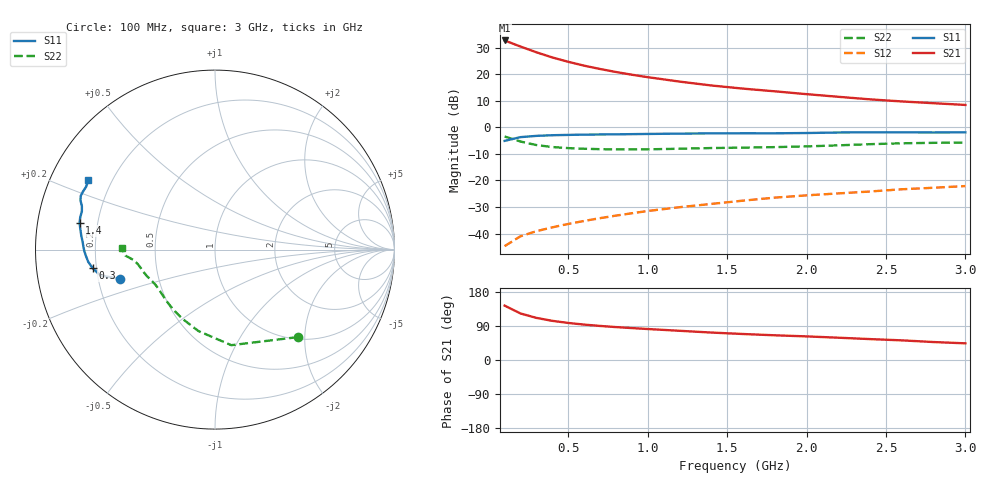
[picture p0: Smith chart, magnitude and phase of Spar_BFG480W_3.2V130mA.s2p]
! Filename: 3_2130BFG480.001
! Title: BFG480W
! Bias: Vce=3.2V; Ic=130mA
! Company: NXP Semiconductors NL
! User: Quality&Reliability T&D
! Measure time: 10 Nov 1999 / 11:58:35
#  MHz  S  MA  R 50
! Freq  S11  S21  S12  S22  :
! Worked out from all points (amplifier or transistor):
!   20 points, 100 MHz to 3 GHz, reference 50 ohm
!   highest |S21| = 32.7 dB at 100 MHz (marker M1)
!   |S21| within 3 dB of that: start of sweep to 232.7 MHz
!   unconditionally stable (mu >= 1): 528.6 MHz to end of sweep
!   at 400 MHz: K = 0.92, MSG = 31.9 dB, |S12| = -37.6 dB
!   at 1.2 GHz: K = 1.11, MAG = 21.6 dB, |S12| = -30.1 dB
!   at 3 GHz: K = 1.08, MAG = 13.6 dB, |S12| = -22.1 dB
!   S11 on the Smith chart (normalised r, x): 100 MHz: 0.29, -0.14; 300 MHz: 0.18, -0.07; 1.4 GHz: 0.13, +0.10; 3 GHz: 0.12, +0.25
100  0.5557 -163.0  42.95 143.5  0.005819 67.8  0.671 -46.6
200  0.6532 -167.2  32.97 122.8  0.008943 61.0  0.5402 -80.3
300  0.6899 -171.4  25.75 111.1  0.01113 61.4  0.4634 -101.4
400  0.7096 -174.5  20.58 103.4  0.01315 63.8  0.4257 -115.4
500  0.7196 -177.1  17.06 97.8  0.01521 66.1  0.4062 -125.2
600  0.728 -179.3  14.43 93.4  0.01734 68.0  0.395 -132.3
700  0.7331 178.8  12.5 89.9  0.01954 70.1  0.388 -137.7
800  0.7378 177.0  10.97 86.9  0.02184 71.6  0.3841 -142.2
900  0.7437 175.3  9.75 84.3  0.0242 73.2  0.3833 -146.0
1000  0.7499 173.8  8.774 81.8  0.02668 73.9  0.3852 -149.4
1200  0.7604 171.0  7.238 77.1  0.03141 75.2  0.3952 -154.8
1400  0.769 168.8  6.122 72.4  0.03623 75.8  0.4073 -158.8
1600  0.7722 166.5  5.341 68.6  0.04174 76.3  0.415 -161.9
1800  0.7716 164.0  4.749 65.2  0.04759 76.6  0.424 -165.4
2000  0.7804 161.9  4.202 62.3  0.0525 77.0  0.4373 -169.3
2200  0.7985 159.9  3.746 58.8  0.05711 76.8  0.4578 -172.7
2400  0.8058 158.1  3.353 55.2  0.06208 76.1  0.4817 -174.8
2600  0.8036 156.3  3.063 51.8  0.06837 75.3  0.5005 -176.2
2800  0.7991 154.0  2.838 47.4  0.07302 73.8  0.5103 -177.9
3000  0.8035 151.4  2.634 44.0  0.07849 72.9  0.5185 179.2
